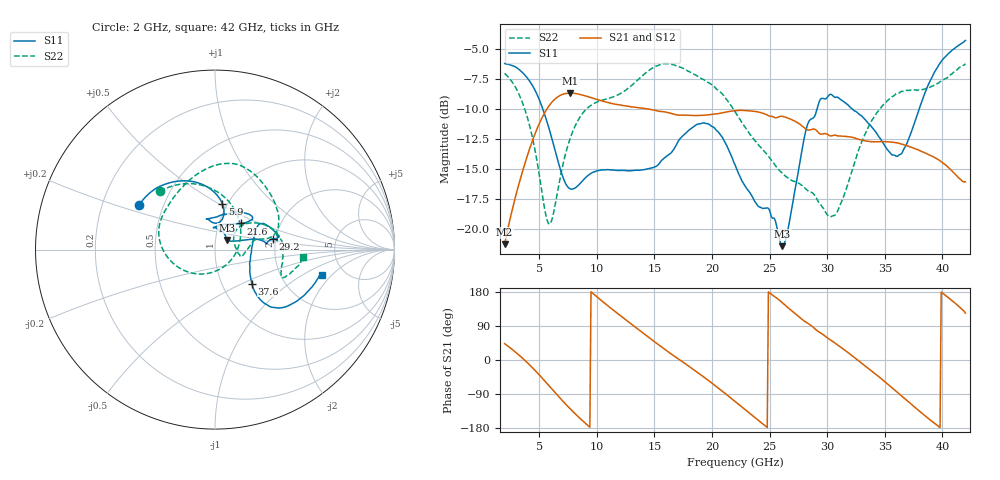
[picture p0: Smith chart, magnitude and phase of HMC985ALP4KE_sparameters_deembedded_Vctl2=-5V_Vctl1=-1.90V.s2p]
!s2p File: Measurements: S11, S21, S12, S22
# GHz S dB R 50.0
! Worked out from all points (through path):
!   401 points, 2 GHz to 42 GHz, reference 50 ohm
!   highest |S21| = -8.65 dB at 7.7 GHz (marker M1); lowest = -21.3 dB at 2 GHz (marker M2)
!   lowest |S11| = -21.4 dB at 26.1 GHz (marker M3), VSWR 1.19, Z = 56.7 + j6.15 ohm
!   |S11| at or under -10 dB: 5.327 GHz to 29.11 GHz (23.79 GHz wide, 138 % of centre); 32.22 GHz to 37.98 GHz (5.757 GHz wide, 16.4 % of centre)
!   |S22| runs from -19.6 to -6.2 dB; largest |S21 - S12| = 0.00037
!   S11 on the Smith chart (normalised r, x): 2 GHz: 0.36, +0.24; 5.9 GHz: 0.95, +0.52; 21.6 GHz: 1.28, +0.39; 29.2 GHz: 1.92, +0.26; 37.6 GHz: 1.38, -0.57; 42 GHz: 3.39, -1.55
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2  -6.18 149.4  -21.25 43.2  -21.26 43.2  -7.00 133.5
3.2  -6.63 130.3  -16.36 14.3  -16.37 14.3  -8.64 102.8
4.4  -7.98 108.1  -12.66 -19.9  -12.66 -19.9  -12.28 62.1
5.9  -11.74 80.9  -9.65 -69.5  -9.65 -69.5  -19.57 -48.2
7.7  -16.63 86.4  -8.65 -129.1  -8.65 -129.1  -12.39 -159.8
8.7  -16.02 98.3  -8.80 -158.4  -8.80 -158.4  -10.42 175.6
10.2  -15.09 103.7  -9.23 162.0  -9.23 162.0  -9.32 153.4
12.2  -15.09 105.7  -9.67 113.5  -9.68 113.5  -8.60 128.0
15.4  -14.54 84.0  -10.16 39.5  -10.16 39.6  -6.31 82.8
18.3  -11.52 49.6  -10.51 -23.1  -10.52 -23.1  -7.00 50.1
21.6  -13.70 44.9  -10.16 -99.5  -10.16 -99.5  -9.60 13.1
22  -14.62 50.7  -10.11 -109.4  -10.12 -109.4  -10.19 12.1
24.1  -18.14 91.3  -10.23 -161.0  -10.24 -161.0  -13.04 13.1
26.1  -21.40 39.3  -10.59 151.3  -10.59 151.3  -15.32 -3.5
28.7  -10.77 6.3  -11.66 88.7  -11.66 88.7  -16.94 -12.5
29.2  -9.70 10.7  -11.89 75.7  -11.90 75.8  -17.64 -8.9
30.7  -9.00 13.3  -12.16 44.2  -12.16 44.2  -18.80 24.4
32.3  -10.07 26.6  -12.36 8.2  -12.37 8.2  -14.70 42.9
35.4  -13.54 7.3  -12.71 -67.3  -12.71 -67.3  -9.15 17.2
37.6  -11.09 -42.6  -13.26 -124.4  -13.27 -124.4  -8.38 -5.7
39.8  -6.15 -41.1  -14.29 -178.3  -14.29 -178.2  -7.70 -22.2
42  -4.26 -13.5  -16.03 123.6  -16.04 123.6  -6.20 -5.1
